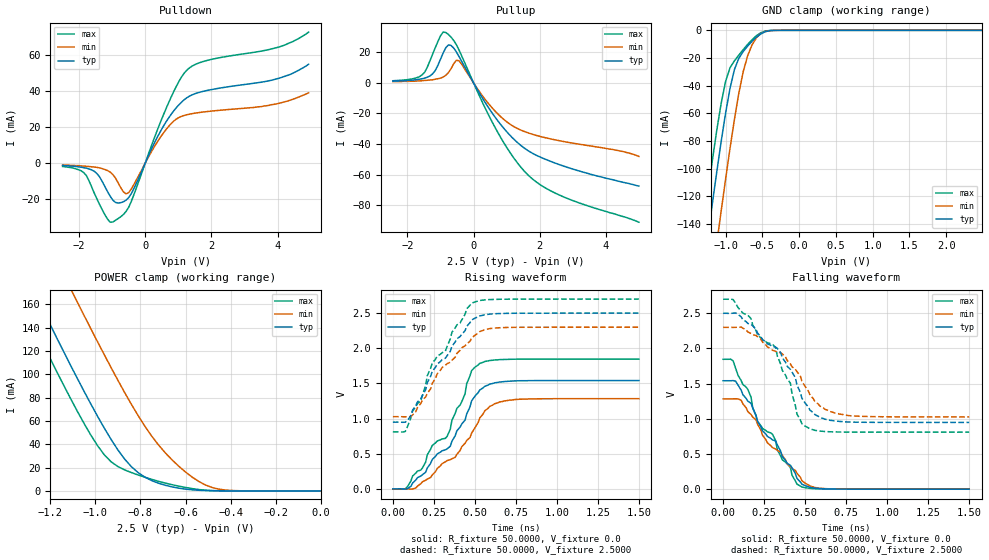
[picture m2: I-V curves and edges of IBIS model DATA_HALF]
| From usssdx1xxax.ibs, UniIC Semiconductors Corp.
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|   Model DATA_HALF
[Model]  DATA_HALF
Model_type   I/O
Polarity   Non-Inverting
Enable   Active-High
Vinl =   940.000mV
Vinh =   1.560V
Vmeas =   1.250V
Vref =   1.250V
Cref =   30.000pF
Rref =   50.000Ohm
C_comp   2.2640pF   2.2480pF   2.2810pF
[Temperature Range]   25.0000   0.1250k   -55.0000
[Voltage Range]   2.5000V   2.3000V   2.7000V
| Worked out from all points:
|   slope of the pulldown table from 0 to 0.375 V, typ, clamps not added: 25.4 ohm
|   slope of the pullup table from 0 to 0.375 V, typ, clamps not added: 27.5 ohm
|   GND clamp passes 1 mA (typ) near -0.46 V on its own axis
|   POWER clamp passes 1 mA (typ) near -0.57 V on its own axis
|   rising waveform, R_fixture 50.0000, V_fixture 0.0: 20-80 % time 265ps typ, 273ps min, 252ps max; typ from 0 V to 1.54 V
|   rising waveform, R_fixture 50.0000, V_fixture 2.5000: 20-80 % time 256ps typ, 256ps min, 243ps max; typ from 0.949 V to 2.5 V
|   falling waveform, R_fixture 50.0000, V_fixture 0.0: 20-80 % time 257ps typ, 263ps min, 260ps max; typ from 1.54 V to 0 V
|   falling waveform, R_fixture 50.0000, V_fixture 2.5000: 20-80 % time 269ps typ, 289ps min, 257ps max; typ from 2.5 V to 0.949 V
[Pulldown]
|Voltage   I(typ)   I(min)   I(max)
-2.5V     -1.3mA     -1.1mA     -1.9mA
-1.86V    -2.6mA     -1.7mA     -5.3mA
-1.46V    -5.9mA     -2.4mA     -20mA
-1.14V    -15.9mA    -4.2mA     -31.2mA
-980mV    -20.63mA   -6.4mA     -32.81mA
-660mV    -21.54mA   -16.05mA   -28.6mA
-500mV    -19.2mA    -16.4mA    -24.57mA
540mV     20.23mA    16.51mA    26.4mA
1.26V     36.38mA    26.9mA     51.76mA
1.9V      40.53mA    28.73mA    57.26mA
4.06V     47.3mA     33.3mA     64.7mA
4.94V     55mA       39.1mA     72.9mA
[Pullup]
|Voltage   I(typ)   I(min)   I(max)
-2.44V    1.1mA      800uA      1.4mA
-1.56V    2.7mA      1.4mA      5.2mA
-1.16V    8mA        2.4mA      22.88mA
-1V       15.46mA    3.1mA      30.75mA
-840mV    22.97mA    4.97mA     32.96mA
-680mV    24.48mA    9.33mA     29.92mA
-440mV    17.23mA    14.5mA     21.51mA
680mV     -23.26mA   -19.12mA   -30.33mA
1.16V     -35.58mA   -27.83mA   -47.38mA
1.64V     -44.21mA   -32.62mA   -60.08mA
2.68V     -54.09mA   -38.17mA   -74.16mA
5V        -67.5mA    -48.1mA    -91.1mA
[GND_clamp]
|Voltage   I(typ)   I(min)   I(max)
-2.5V     -683.1mA   -736.1mA   -653.6mA
-1.3V     -173.1mA   -226.8mA   -141.1mA
-1.24V    -149mA     -202.4mA   -117.2mA
-1.18V    -125.4mA   -178.1mA   -94.12mA
-1.12V    -102.4mA   -154.2mA   -72.32mA
-1.06V    -80.41mA   -130.7mA   -52.79mA
-1V       -59.95mA   -107.7mA   -37.03mA
-880mV    -28.39mA   -64.58mA   -22.05mA
-760mV    -15.32mA   -29.84mA   -13.95mA
-700mV    -11.37mA   -18.38mA   -10.19mA
-520mV    -2.567mA   -2.292mA   -1.702mA
2.48V     19.82nA    1.016uA    2.464nA
[POWER_clamp]
|Voltage   I(typ)   I(min)   I(max)
-2.49V    671mA      736.6mA    644.5mA
-1.35V    201.6mA    268.3mA    172.7mA
-1.32V    189.6mA    256.3mA    160.6mA
-1.26V    165.8mA    232.4mA    136.8mA
-1.11V    107.6mA    173.4mA    79.15mA
-1.08V    96.37mA    161.8mA    68.24mA
-960mV    53.65mA    116.5mA    30.86mA
-840mV    20.7mA     74.06mA    15.7mA
-720mV    6.602mA    39.33mA    8.242mA
-600mV    1.533mA    16.16mA    2.964mA
-450mV    76.58uA    1.436mA    135uA
0V        21.05nA    42.84nA    5.083nA
[Ramp]
| variable   typ   min   max
dV/dt_r  0.9246/0.2643n   0.7698/0.2705n   1.1076/0.2553n
dV/dt_f  0.9306/0.2690n   0.7638/0.2830n   1.1339/0.2530n
R_load = 50.0000
[Rising Waveform]
R_fixture= 50.0000
V_fixture= 0.0
V_fixture_min= 0.0
V_fixture_max= 0.0
|time   V(typ)   V(min)   V(max)
0s        0V         0V         0V
75.76ps   -4.006mV   375.5uV    -1.288mV
180ps     200.9mV    100.8mV    296.4mV
240ps     418.2mV    198.3mV    617.9mV
330ps     568.4mV    402.5mV    744.4mV
440ps     978.5mV    647.8mV    1.351V
480ps     1.251V     791.8mV    1.681V
530ps     1.407V     1.01V      1.785V
710ps     1.532V     1.262V     1.843V
1.5ns     1.541V     1.283V     1.846V
[Rising Waveform]
R_fixture= 50.0000
V_fixture= 2.5000
V_fixture_min= 2.3000
V_fixture_max= 2.7000
|time   V(typ)   V(min)   V(max)
0s        949mV      1.027V     810.1mV
75.76ps   948.9mV    1.025V     817.2mV
120ps     1.12V      1.052V     1.104V
170ps     1.279V     1.214V     1.25V
240ps     1.672V     1.501V     1.79V
320ps     1.859V     1.757V     1.959V
360ps     2.029V     1.829V     2.227V
480ps     2.402V     2.144V     2.641V
620ps     2.491V     2.288V     2.696V
1.5ns     2.5V       2.3V       2.7V
[Falling Waveform]
R_fixture= 50.0000
V_fixture= 0.0
V_fixture_min= 0.0
V_fixture_max= 0.0
|time   V(typ)   V(min)   V(max)
0s        1.541V     1.283V     1.846V
60.61ps   1.543V     1.284V     1.824V
110ps     1.406V     1.263V     1.542V
170ps     1.22V      1.061V     1.307V
210ps     961.6mV    921.8mV    959.9mV
300ps     701.4mV    591.2mV    782.3mV
360ps     465.4mV    480mV      418.3mV
480ps     70.89mV    120.7mV    30.38mV
620ps     4.617mV    7.423mV    1.94mV
1.5ns     -719.4nV   0V         0V
[Falling Waveform]
R_fixture= 50.0000
V_fixture= 2.5000
V_fixture_min= 2.3000
V_fixture_max= 2.7000
|time   V(typ)   V(min)   V(max)
0s        2.5V       2.3V       2.7V
60.61ps   2.501V     2.299V     2.695V
210ps     2.217V     2.166V     2.194V
320ps     2.019V     1.959V     2.014V
360ps     1.871V     1.923V     1.69V
410ps     1.702V     1.78V      1.506V
450ps     1.479V     1.67V      1.068V
530ps     1.121V     1.334V     854.8mV
740ps     957.2mV    1.053V     811.3mV
1.5ns     949mV      1.027V     810.1mV
